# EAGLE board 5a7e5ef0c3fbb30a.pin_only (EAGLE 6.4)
REV: A

Size 50.8 x 22.86 mm. Coordinates in mm from the lower left corner, seen from the top.
Outline: 2.54,0 48.26,0 arc90 50.8,2.54 50.8,3.81 49.91,4.7 49.91,15.62 50.8,16.51 50.8,20.32 arc90 48.26,22.86 2.54,22.86 arc90 0,20.32 0,13.97 0.51,13.46 0.51,9.4 0,8.89 0,2.54 arc90 2.54,0
Copper layers (1*16): Top 0.035mm / dielectric 1.5mm / Bottom 0.035mm
Design rules "adafruit *": minimum track width 8mil, minimum drill 15.5mil, track to track 8mil, track to pad 8mil, pad to pad 8mil, via to via 8mil, smd to smd 8mil, copper to edge 10mil, drill to drill 8mil, minimum pad ring 10mil, minimum via ring 8mil, stop-mask expansion 2mil, vias tented up to drill 20mil, thermal gap 10mil
Holes 2.54 mm at 48.26,20.32 48.26,2.54
tRestrict: area 21.3,6.9 to 21.7,9.7; area 22.1,12.1 to 27.1,12.4; area 26.5,9.7 to 27.1,12.2

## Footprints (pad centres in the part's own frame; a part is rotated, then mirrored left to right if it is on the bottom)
0603-NO = smd 1.1 x 1: 1 -0.85,0; 2 0.85,0
0805-NO = smd 1.3 x 1.5: 1 -0.95,0; 2 0.95,0
CHIPLED_0805_NOOUTLINE = smd 1.2 x 1.2: A 0,-1.05; C 0,1.05
SOD-123 = smd 1.4 x 1.4: A 1.85,0; C -1.85,0
1X16_ROUND = drill 1 pad 1.676: 1 -19.05,0; 2 -16.51,0; 3 -13.97,0; 4 -11.43,0; 5 -8.89,0; 6 -6.35,0; 7 -3.81,0; 8 -1.27,0; 9 1.27,0; 10 3.81,0; 11 6.35,0; 12 8.89,0; 13 11.43,0; 14 13.97,0; 15 16.51,0; 16 19.05,0
1X12_ROUND = drill 1 pad 1.676: 1 -13.97,0; 2 -11.43,0; 3 -8.89,0; 4 -6.35,0; 5 -3.81,0; 6 -1.27,0; 7 1.27,0; 8 3.81,0; 9 6.35,0; 10 8.89,0; 11 11.43,0; 12 13.97,0
KMR2 = smd 1 x 1: 1 2,0.8; 2 2,-0.8; 3 -2,0.8; 4 -2,-0.8
TESTPOINT_ROUND_1.5MM = smd 1.5 x 1.5: P$1 0,0
SOT23-5 = smd 0.55 x 1.2: 1 -0.95,-1.3; 2 0,-1.3; 3 0.95,-1.3; 4 0.95,1.3; 5 -0.95,1.3
TQFN48_7MM = smd 0.25 x 0.75: 1 -2.75,-3.475; 2 -2.25,-3.475; 3 -1.75,-3.475; 4 -1.25,-3.475; 5 -0.75,-3.475; 6 -0.25,-3.475; 7 0.25,-3.475; 8 0.75,-3.475; 9 1.25,-3.475; 10 1.75,-3.475; 11 2.25,-3.475; 12 2.75,-3.475; 25 2.75,3.475; 26 2.25,3.475; 27 1.75,3.475; 28 1.25,3.475; 29 0.75,3.475; 30 0.25,3.475; 31 -0.25,3.475; 32 -0.75,3.475; 33 -1.25,3.475; 34 -1.75,3.475; 35 -2.25,3.475; 36 -2.75,3.475 | smd 0.75 x 0.25: 13 3.475,-2.75; 14 3.475,-2.25; 15 3.475,-1.75; 16 3.475,-1.25; 17 3.475,-0.75; 18 3.475,-0.25; 19 3.475,0.25; 20 3.475,0.75; 21 3.475,1.25; 22 3.475,1.75; 23 3.475,2.25; 24 3.475,2.75; 37 -3.475,2.75; 38 -3.475,2.25; 39 -3.475,1.75; 40 -3.475,1.25; 41 -3.475,0.75; 42 -3.475,0.25; 43 -3.475,-0.25; 44 -3.475,-0.75; 45 -3.475,-1.25; 46 -3.475,-1.75; 47 -3.475,-2.25; 48 -3.475,-2.75 | smd 4.7 x 4.7: THERMAL 0,0
MOUNTINGHOLE_2.5_PLATED = drill 2.5 pad 3.2: P$1 0,0
FIDUCIAL_1MM = smd 1 x 1: 1 0,0
JSTPH2 = smd 1 x 4.6: 1 -1,-3.7; 2 1,-3.7 | smd 1.6 x 3.4: NC1 -3.4,1.5; NC2 3.4,1.5
XTAL3215 = smd 1.1 x 1.9: P$1 1.2,0; P$2 -1.2,0
4UCONN_20329_V2 = smd 1 x 2: BASE@1 -0.75,-2; BASE@2 0.75,-2 | smd 0.4 x 1.35: D+ 0,0.775; D- -0.65,0.775; GND 1.3,0.775; ID 0.65,0.775; VBUS -1.3,0.775 | drill 0.8 pad 1.2 offset: SPRT@1 -3.3,0.9; SPRT@2 3.3,0.9 | drill 0.9 pad 2.5 square: SPRT@3 -3.6,-1.9; SPRT@4 3.6,-1.9 | hole 0.7: -1.95,0; 1.95,0
MICROSD = smd 0.7 x 1.5: 1 9,-10.64; 2 7.9,-10.24; 3 6.8,-10.64; 4 5.7,-11.04; 5 4.6,-10.64; 6 3.5,-11.04; 7 2.4,-10.64; 8 1.3,-10.64 | smd 1.8 x 1.4: CD1 2,-0.44; CD2 8,-0.44 | smd 1.4 x 1.9: MT1 0.4,-13.54; MT2 13.6,-14.44

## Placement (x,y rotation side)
C1  1uF  [0603-NO]  17.78,11.81 90 top
C2  22pF  [0603-NO]  17.65,7.49 90 top
C3  10µF  [0805-NO]  11.43,11.18 270 top
C4  22pF  [0603-NO]  16.38,7.49 90 top
C5  10uF  [0805-NO]  31.62,13.84 270 top
C6  10µF  [0805-NO]  8.09,12.96 90 top
C7  1uF  [0603-NO]  16.4,11.86 90 top
C8  10µF  [0805-NO]  13.86,11.62 270 top
C14  1uF  [0603-NO]  10.72,4.34 0 top
CHG  ORANGE  [CHIPLED_0805_NOOUTLINE]  2.41,5.59 270 top
D1  MBR120  [SOD-123]  17.78,18.67 180 top
JP1  [1X16_ROUND]  25.4,1.27 180 top
JP3  [1X12_ROUND]  30.48,21.59 0 top
L  RED  [CHIPLED_0805_NOOUTLINE]  2.65,17.36 90 top
L1  GREEN  [CHIPLED_0805_NOOUTLINE]  30.48,4.57 270 top
R1  100k  [0603-NO]  15.62,16.13 90 top
R2  1K  [0603-NO]  6.1,4.32 0 top
R3  100k  [0603-NO]  22.35,18.54 0 top
R4  1K  [0603-NO]  30.86,5.97 180 top
R6  100K  [0603-NO]  22.48,17.27 180 top
R7  2.2K  [0603-NO]  5.71,20.95 270 top
R8  10K\  [0603-NO]  13.84,4.32 180 top
SW1  SPST_TACT-KMR2  [KMR2]  9.4,6.48 180 top
TP1  [TESTPOINT_ROUND_1.5MM]  15.37,5.33 0 bottom
TP2  [TESTPOINT_ROUND_1.5MM]  17.91,5.33 0 bottom
U2  SPX3819-3.3  [SOT23-5]  18.16,15.49 180 top
U3  MCP73831T-2ACI/OT  [SOT23-5]  13.84,7.75 180 top
U$4  ATSAMD21G18_QFN  [TQFN48_7MM]  24.13,9.65 0 top
U$7  [ADAFRUIT_3.5MM]  33.15,7.11 90 top
U$9  [PCBFEAT-REV-040]  29.08,14.48 0 top
U$13  [FEATHERLOGO]  33.15,10.54 0 bottom
U$14  [ADALOGGER_LOGO]  35.69,6.73 0 bottom
U$31  MOUNTINGHOLE2.5  [MOUNTINGHOLE_2.5_PLATED]  2.54,20.32 270 top
U$32  MOUNTINGHOLE2.5  [MOUNTINGHOLE_2.5_PLATED]  2.54,2.54 270 top
U$34  FIDUCIAL""  [FIDUCIAL_1MM]  10.79,20.07 270 top
U$35  FIDUCIAL""  [FIDUCIAL_1MM]  46.4,0.77 270 top
X1  JSTPH  [JSTPH2]  10.79,19.3 0 top
X2  32.768  [XTAL3215]  17.65,4.83 0 top
X3  microUSB  [4UCONN_20329_V2]  4.45,11.43 270 top
X4  microsd  [MICROSD]  33.91,4.45 90 top

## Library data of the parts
C1-C7 C14 CHG D1 JP1 JP3 L L1 R1-R4 R6-R8 TP1 TP2 U2 U3 U$4 U$7 U$9 U$13 U$14 X1 X3 X4 = microbuilder
C8 = microbuilder; COMPANY: ADAFRUIT INDUSTRIES; DRAWN: KTOWN; REV: A
SW1 = adafruit
U$31 U$32 U$34 U$35 = microbuilder; BOM: EXCLUDE
X2 = adafruit2

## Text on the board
tPlace: BAT | En | USB | 13 | 12 | 11 | ~ | 10 | ~ | 9 | ~ | 6 | ~5 | SCL | SDA | #13 | Feather M0 / Adalogger | adafruit! | RST | CHG | #8 | RX | 0 | TX | 1 | GND | RST | 3V | ARf | GND | A0 | A1 | A2 | A3 | A4 | A5 | SCK | MOSI | MISO
bPlace: 3.7/4.2V / LiPoly Batt / µUSB charge | BAT | En | 13 | 12 | 6 | ~ | 5 | SCL | SDA | USB | 11~ | 10~ | 9~ | 21 | 20 | uSD card uses: / MISO/MOSI/SCK (SPI) / 4 (CS) & 7 (CD) | Feather M0 / uSD Adalogger | ATSAMD21G18 / 48MHz & 3.3V | swclk | swdio | ARef | GND | SCK | 24 | MOSI | 23 | MISO | 22 | 0 | 1 | RST | 3V | A0 | A1 | A2 | A3 | A4 | A5 | RX | TX | GND

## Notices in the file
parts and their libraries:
microbuilder: This work is placed in the public domain, and may be freely used for commercial and non-commercial work with the following conditions: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
